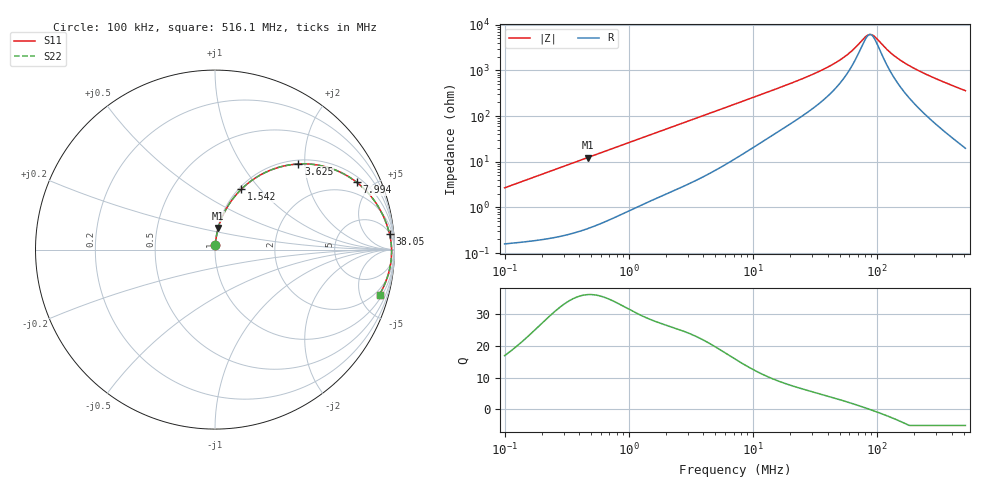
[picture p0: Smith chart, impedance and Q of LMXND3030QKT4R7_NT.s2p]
! LMXND3030QKT4R7_NT  S-PARAMETER MODEL  ( Standard Model )
! Model Generated by TAIYO YUDEN Corporation (https://www.yuden.co.jp/en/)
! Version 1.0
! TAIYO YUDEN Control No. 20250724
! Copyright(c) 2025 TAIYO YUDEN CO.,LTD. All Rights Reserved.
! Product Description (link to TY-COMPAS)
! https://ds.yuden.co.jp/TYCOMPAS/or/detail?pn=LMXND3030QKT4R7MNT&u=M
! Products Name : Inductors
! Characteristics :
!  Inductance : 4.7 [uH] , SRF(min) : 40 [MHz] , DC Resistance(max) : 0.144 [Ohm]
!  Rated Current : Saturation  1020 [m A] , Temp Rise  1600 [m A] (40 [degC])
!  Case Size : 3.0 x 3.0 / 0.118 x 0.118 [mm/inch] , Thickness : 1.5 / 0.059 [mm/inch]
!  (Conditions: Temperature = 25 [degC] , DC Bias Current = 0 [A])
! External Node Assignments :
!  1  o---GGG---o  2
! GND o---------o GND
! Frequency Range : 0.1MHz  -  516.089782MHz  [ 402 STEP ]
# MHz S RI R 50
! Freq[MHz].  S11 Real  S11 Imag  S21 Real  S21 Imag  S12 Real  S12 Imag  S22 Real  S22 Imag
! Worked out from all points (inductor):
!   401 points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, 100 kHz to 516.1 MHz, reference 50 ohm
!   read as one part in series: L = 4.25 uH near 104.4 kHz
!   highest Q = 36 at 465.9 kHz (marker M1), where L = 4.21 uH
!   self-resonance near 87.92 MHz
!   S11 on the Smith chart (normalised r, x): 100 kHz: 1.00, +0.05; 1.542 MHz: 1.03, +0.80; 3.625 MHz: 1.08, +1.86; 7.994 MHz: 1.28, +4.07; 38.05 MHz: 6, +21; 516.1 MHz: 1.39, -7.19
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0.1  0.00229 0.0266  0.9977 -0.0266  0.9977 -0.0266  0.00229 0.0266
0.418679  0.0151 0.1088  0.9849 -0.1088  0.9849 -0.1088  0.0151 0.1088
0.465898  0.0182 0.1205  0.9818 -0.1205  0.9818 -0.1205  0.0182 0.1205
0.923227  0.0617 0.2257  0.9383 -0.2257  0.9383 -0.2257  0.0617 0.2257
1.541956  0.1473 0.337  0.8527 -0.337  0.8527 -0.337  0.1473 0.337
1.752923  0.1803 0.3665  0.8197 -0.3665  0.8197 -0.3665  0.1803 0.3665
3.625305  0.4652 0.4771  0.5348 -0.4771  0.5348 -0.4771  0.4652 0.4771
4.995418  0.6143 0.462  0.3857 -0.462  0.3857 -0.462  0.6143 0.462
7.183939  0.7568 0.3986  0.2432 -0.3986  0.2432 -0.3986  0.7568 0.3986
7.994139  0.7903 0.3745  0.2097 -0.3745  0.2097 -0.3745  0.7903 0.3745
13.93474  0.9053 0.2465  0.0947 -0.2465  0.0947 -0.2465  0.9053 0.2465
30.07766  0.9651 0.1146  0.0349 -0.1146  0.0349 -0.1146  0.9651 0.1146
38.04907  0.973 0.085  0.027 -0.085  0.027 -0.085  0.973 0.085
55.90063  0.9806 0.0433  0.0194 -0.0433  0.0194 -0.0433  0.9806 0.0433
80.39102  0.9837 0.00838  0.0163 -0.00838  0.0163 -0.00838  0.9837 0.00838
85.71424  0.9839 0.00238  0.0161 -0.00238  0.0161 -0.00238  0.9839 0.00238
95.38103  0.9841 -0.00765  0.0159 0.00765  0.0159 0.00765  0.9841 -0.00765
125.929  0.9833 -0.0345  0.0167 0.0345  0.0167 0.0345  0.9833 -0.0345
159.3036  0.9812 -0.0592  0.0188 0.0592  0.0188 0.0592  0.9812 -0.0592
214.8676  0.9756 -0.0951  0.0244 0.0951  0.0244 0.0951  0.9756 -0.0951
329.4634  0.9583 -0.1599  0.0417 0.1599  0.0417 0.1599  0.9583 -0.1599
516.0898  0.9165 -0.2505  0.0835 0.2505  0.0835 0.2505  0.9165 -0.2505
